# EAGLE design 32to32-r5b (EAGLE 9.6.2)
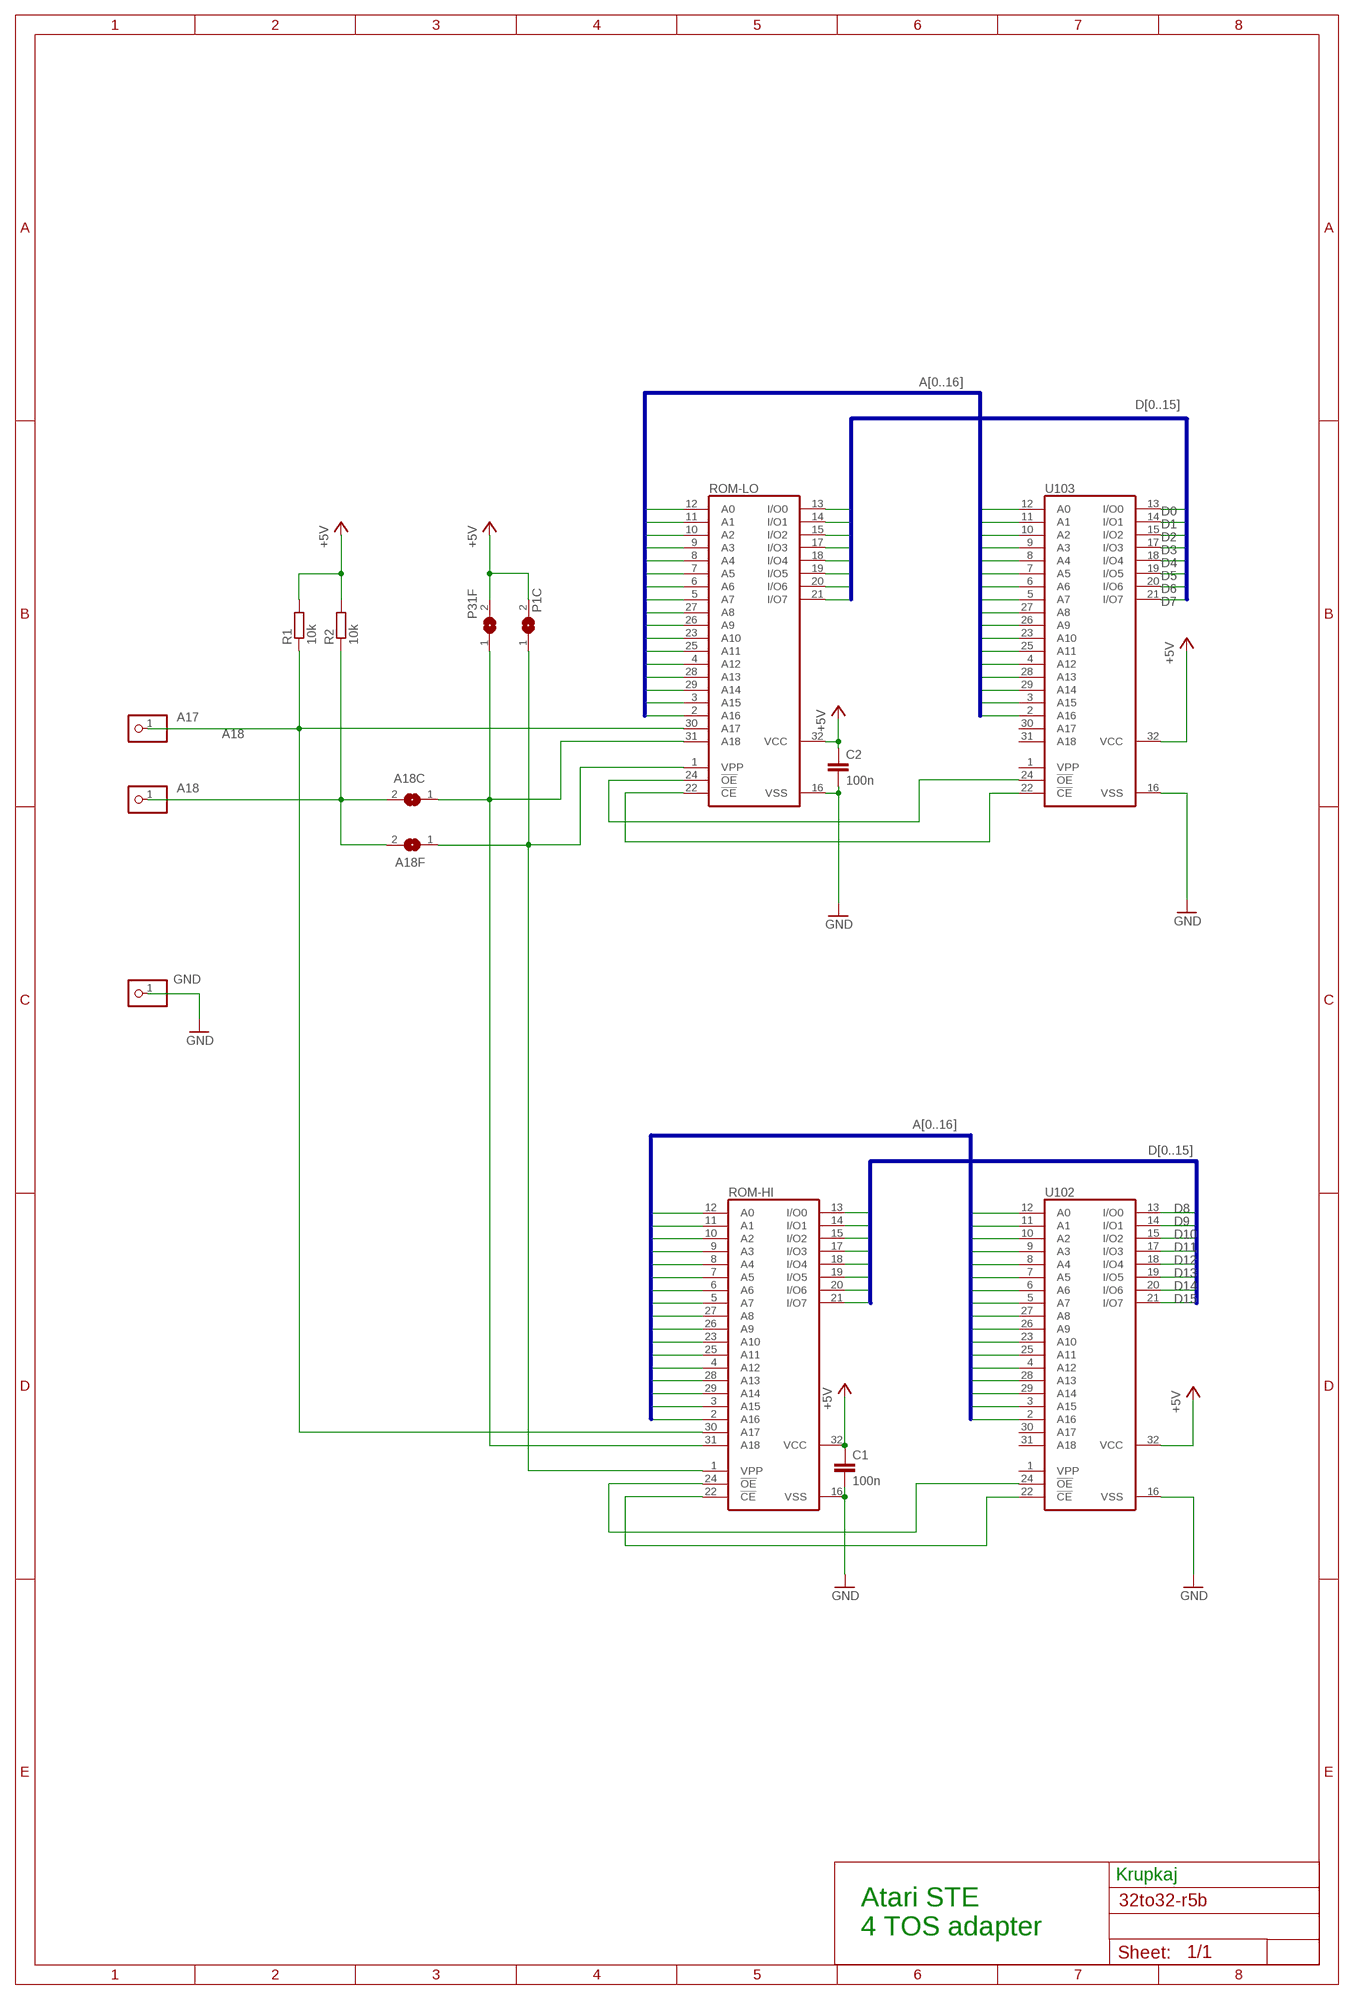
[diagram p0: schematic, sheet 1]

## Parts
A17  PINHD-1X1  [1X01]
A18  PINHD-1X1  [1X01]
A18C  SJ  [SJ]
A18F  SJ  [SJ]
C1  100n  C-EUC0805K  [C0805K]
C2  100n  C-EUC0805K  [C0805K]
GND  PINHD-1X1  [1X01]
P1C  SJ  [SJ]
P31F  SJ  [SJ]
R1  10k  R-EU_R0805  [R0805]
R2  10k  R-EU_R0805  [R0805]
ROM-HI  27C4001G  [DIL32]
ROM-LO  27C4001G  [DIL32]
U102  27C4001G  [DIL32]
U103  27C4001G  [DIL32]

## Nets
+5V: C1.1 C2.1 P1C.2 P31F.2 R1.2 R2.2 ROM-HI.32(VCC) ROM-LO.32(VCC) U102.32(VCC) U103.32(VCC)
/CE: ROM-HI.22(!CE) U102.22(!CE)
/OE: ROM-HI.24(!OE) U102.24(!OE)
A0: ROM-HI.12(A0) ROM-LO.12(A0) U102.12(A0) U103.12(A0)
A1: ROM-HI.11(A1) ROM-LO.11(A1) U102.11(A1) U103.11(A1)
A2: ROM-HI.10(A2) ROM-LO.10(A2) U102.10(A2) U103.10(A2)
A3: ROM-HI.9(A3) ROM-LO.9(A3) U102.9(A3) U103.9(A3)
A4: ROM-HI.8(A4) ROM-LO.8(A4) U102.8(A4) U103.8(A4)
A5: ROM-HI.7(A5) ROM-LO.7(A5) U102.7(A5) U103.7(A5)
A6: ROM-HI.6(A6) ROM-LO.6(A6) U102.6(A6) U103.6(A6)
A7: ROM-HI.5(A7) ROM-LO.5(A7) U102.5(A7) U103.5(A7)
A8: ROM-HI.27(A8) ROM-LO.27(A8) U102.27(A8) U103.27(A8)
A9: ROM-HI.26(A9) ROM-LO.26(A9) U102.26(A9) U103.26(A9)
A10: ROM-HI.23(A10) ROM-LO.23(A10) U102.23(A10) U103.23(A10)
A11: ROM-HI.25(A11) ROM-LO.25(A11) U102.25(A11) U103.25(A11)
A12: ROM-HI.4(A12) ROM-LO.4(A12) U102.4(A12) U103.4(A12)
A13: ROM-HI.28(A13) ROM-LO.28(A13) U102.28(A13) U103.28(A13)
A14: ROM-HI.29(A14) ROM-LO.29(A14) U102.29(A14) U103.29(A14)
A15: ROM-HI.3(A15) ROM-LO.3(A15) U102.3(A15) U103.3(A15)
A16: ROM-HI.2(A16) ROM-LO.2(A16) U102.2(A16) U103.2(A16)
A17: A17.1 R1.1 ROM-HI.30(A17) ROM-LO.30(A17)
A18: A18.1 A18C.2 A18F.2 R2.1
D0: ROM-LO.13(I/O0) U103.13(I/O0)
D1: ROM-LO.14(I/O1) U103.14(I/O1)
D2: ROM-LO.15(I/O2) U103.15(I/O2)
D3: ROM-LO.17(I/O3) U103.17(I/O3)
D4: ROM-LO.18(I/O4) U103.18(I/O4)
D5: ROM-LO.19(I/O5) U103.19(I/O5)
D6: ROM-LO.20(I/O6) U103.20(I/O6)
D7: ROM-LO.21(I/O7) U103.21(I/O7)
D8: ROM-HI.13(I/O0) U102.13(I/O0)
D9: ROM-HI.14(I/O1) U102.14(I/O1)
D10: ROM-HI.15(I/O2) U102.15(I/O2)
D11: ROM-HI.17(I/O3) U102.17(I/O3)
D12: ROM-HI.18(I/O4) U102.18(I/O4)
D13: ROM-HI.19(I/O5) U102.19(I/O5)
D14: ROM-HI.20(I/O6) U102.20(I/O6)
D15: ROM-HI.21(I/O7) U102.21(I/O7)
GND: C1.2 C2.2 GND.1 ROM-HI.16(VSS) ROM-LO.16(VSS) U102.16(VSS) U103.16(VSS)
N$1: A18C.1 P31F.1 ROM-HI.31(A18) ROM-LO.31(A18)
N$2: ROM-LO.22(!CE) U103.22(!CE)
N$3: ROM-LO.24(!OE) U103.24(!OE)
VPP: A18F.1 P1C.1 ROM-HI.1(VPP) ROM-LO.1(VPP)
Unconnected: U102.1(VPP) U102.30(A17) U102.31(A18) U103.1(VPP) U103.30(A17) U103.31(A18)

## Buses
D[0..15]
A[0..16]

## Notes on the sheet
- Krupkaj
- Atari STE
  4 TOS adapter

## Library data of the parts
A17 A18 GND = pinhead:PINHD-1X1: PIN HEADER
A18C A18F P1C P31F = jumper:SJ: SMD solder JUMPER
C1 C2 = rcl:C-EU: CAPACITOR, European symbol
R1 R2 = rcl:R-EU_: RESISTOR, European symbol
ROM-HI ROM-LO U102 U103 = memory-hitachi:27C4001G: MEMORY; OC_FARNELL: unknown; OC_NEWARK: unknown

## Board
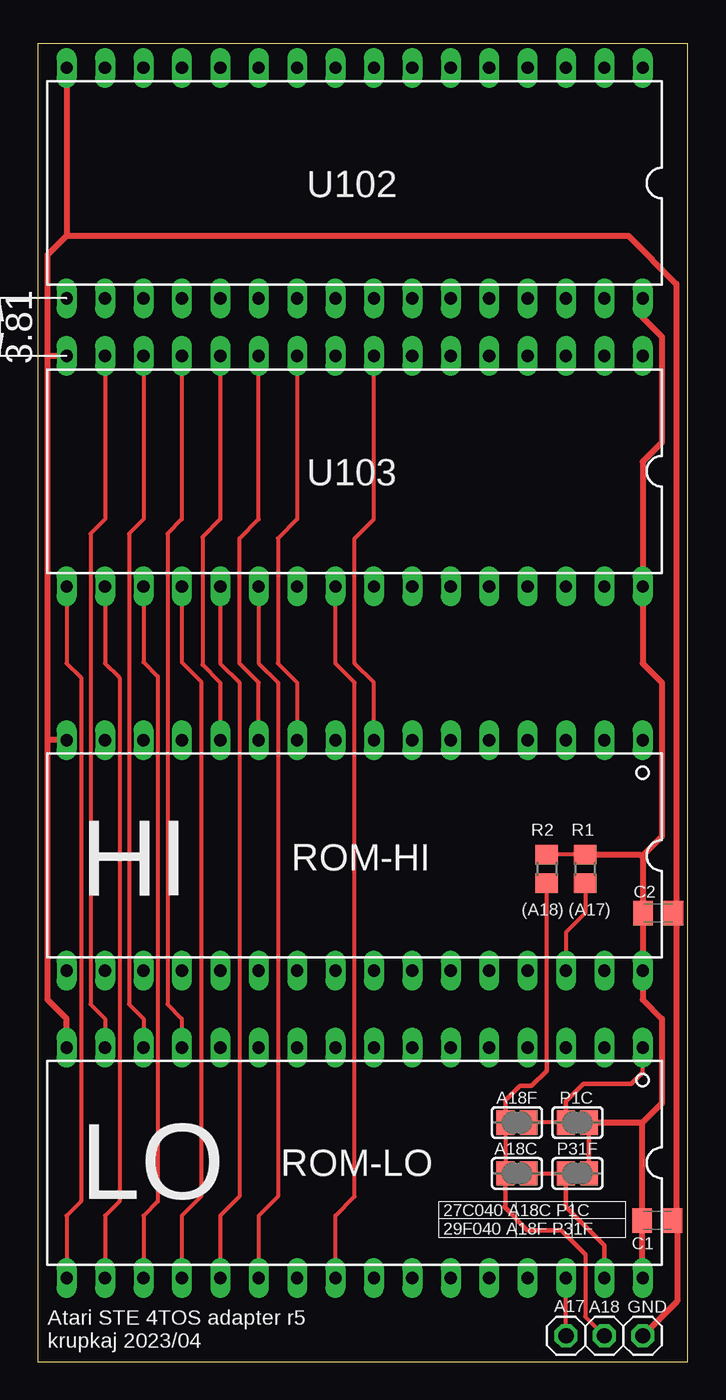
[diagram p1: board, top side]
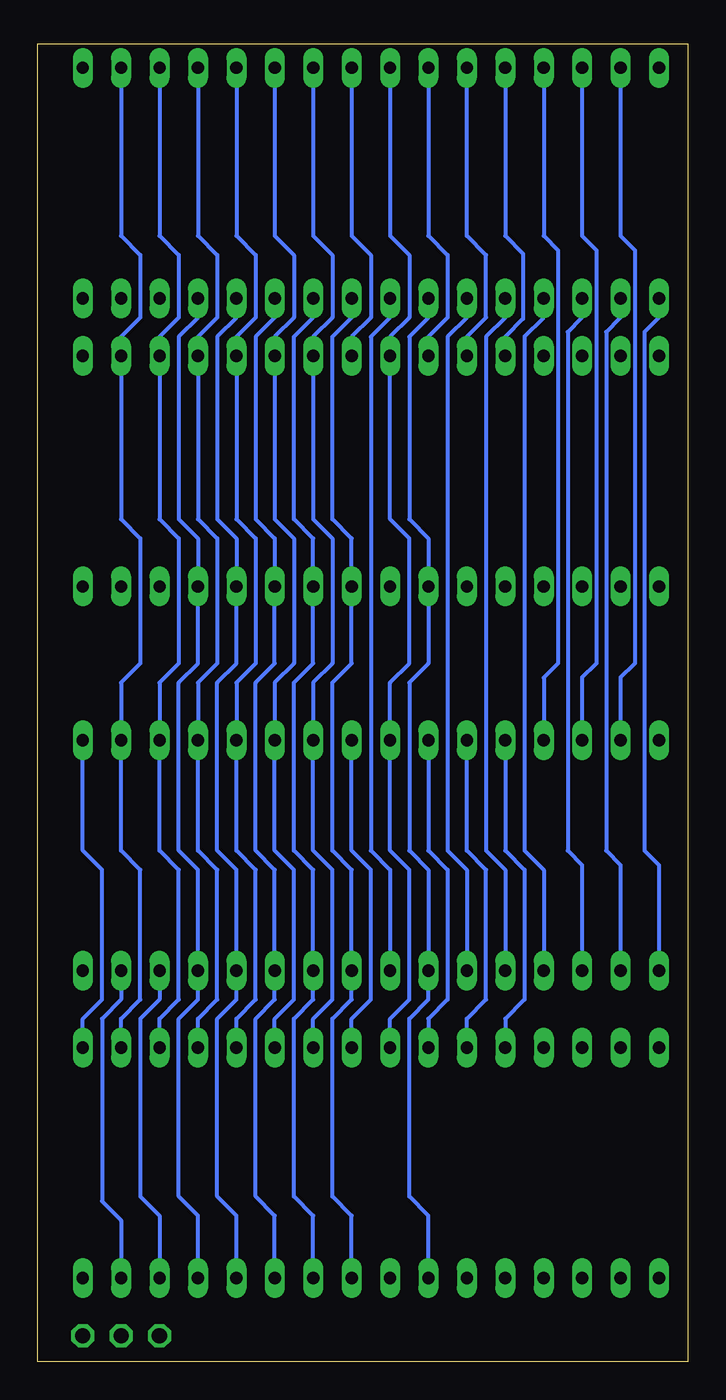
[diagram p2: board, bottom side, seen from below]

Size 42.98 x 87.11 mm. Coordinates in mm from the lower left corner, seen from the top.
Outline: 0,0 42.98,0 42.98,87.11 0,87.11 0,0
Copper layers (1*16): Top 0.035mm / dielectric 1.5mm / Bottom 0.035mm
Design rules "SeeedStudio_2layer_DRU_no_angle_20140221": minimum track width 6mil, minimum drill 12mil, track to track 6mil, track to pad 6mil, pad to pad 6mil, via to via 6mil, smd to smd 0mil, copper to edge 10mil, drill to drill 10mil, minimum pad ring 10mil, minimum via ring 6mil, stop-mask expansion 2mil, vias tented up to drill 100mil, thermal gap 10mil

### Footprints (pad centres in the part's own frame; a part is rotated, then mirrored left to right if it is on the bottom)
1X01 = drill 1.016 octagon: 1 0,0
SJ = smd 1.168 x 1.6: 1 -0.762,0; 2 0.762,0
C0805K = smd 1.3 x 1.6: 1 -1,0; 2 1,0
R0805 = smd 1.3 x 1.5: 1 -0.95,0; 2 0.95,0
DIL32 = drill 0.813 long: 1 -19.05,-7.62; 2 -16.51,-7.62; 3 -13.97,-7.62; 4 -11.43,-7.62; 5 -8.89,-7.62; 6 -6.35,-7.62; 7 -3.81,-7.62; 8 -1.27,-7.62; 9 1.27,-7.62; 10 3.81,-7.62; 11 6.35,-7.62; 12 8.89,-7.62; 13 11.43,-7.62; 14 13.97,-7.62; 15 16.51,-7.62; 16 19.05,-7.62; 17 19.05,7.62; 18 16.51,7.62; 19 13.97,7.62; 20 11.43,7.62; 21 8.89,7.62; 22 6.35,7.62; 23 3.81,7.62; 24 1.27,7.62; 25 -1.27,7.62; 26 -3.81,7.62; 27 -6.35,7.62; 28 -8.89,7.62; 29 -11.43,7.62; 30 -13.97,7.62; 31 -16.51,7.62; 32 -19.05,7.62

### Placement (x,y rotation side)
A17  34.92,1.71 0 top
A18  37.47,1.71 0 top
A18C  31.69,12.45 180 top
A18F  31.69,15.81 180 top
C1  40.96,9.33 0 top
C2  41.02,29.65 0 top
GND  40.01,1.71 0 top
P1C  35.69,15.81 0 top
P31F  35.69,12.45 0 top
R1  36.2,32.58 90 top
R2  33.66,32.58 90 top
ROM-HI  20.96,33.46 180 top
ROM-LO  20.96,13.14 180 top
U102  20.96,77.91 180 top
U103  20.96,58.86 180 top

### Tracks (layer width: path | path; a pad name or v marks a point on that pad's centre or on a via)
+5V
  Top 0.254: R2.2 R1.2 36.2,33.48
  Top 0.305: P1C.2 P31F.2
  Top 0.406: U102.32 40.01,69.02 41.28,67.75 41.28,60.77 40.01,59.5 U103.32 40.01,46.16 41.28,44.89 41.28,34.73 40.02,33.48 40.02,33.34 | 40.02,33.34 C2.1 40.02,25.86 ROM-HI.32 40.01,23.94 41.28,22.67 41.28,17.08 39.96,15.76 | 36.32,12.57 P31F.2 36.85,12.45 | ROM-LO.32 39.96,5.57 C1.1 39.96,15.76 | R1.2 39.83,33.53 40.02,33.34 | P1C.2 39.91,15.81 39.96,15.76
/CE
  Bottom 0.254: ROM-HI.22 14.61,32.51 15.88,33.78 15.88,67.75 14.61,69.02 U102.22
/OE
  Bottom 0.254: U102.24 19.68,69.02 20.96,67.75 20.96,33.78 19.68,32.51 ROM-HI.24
A0
  Top 0.254: U103.12 12.07,55.69 10.88,54.51 10.88,46.08 12.07,44.89 ROM-HI.12
  Bottom 0.254: U102.12 12.07,74.42 10.88,73.24 10.88,68.94 12.07,67.75 U103.12 | ROM-HI.12 12.07,33.78 10.79,32.51 10.79,23.94 12.07,22.67 ROM-LO.12
A1
  Top 0.254: ROM-HI.11 14.61,44.89 13.34,46.16 13.34,54.42 14.61,55.69 U103.11
  Bottom 0.254: ROM-LO.11 14.61,22.67 13.34,23.94 13.34,32.51 14.61,33.78 ROM-HI.11 | U103.11 14.61,67.75 13.34,69.02 13.34,73.15 14.61,74.42 U102.11
A2
  Top 0.254: U103.10 17.14,55.69 15.88,54.42 15.88,46.16 17.14,44.89 ROM-HI.10
  Bottom 0.254: U102.10 17.14,74.42 15.88,73.15 15.88,69.02 17.14,67.75 U103.10 | ROM-HI.10 17.14,33.78 15.88,32.51 15.88,23.94 17.14,22.67 ROM-LO.10
A3
  Bottom 0.254: U102.9 19.68,74.42 18.42,73.15 18.42,69.02 19.68,67.75 U103.9 19.68,55.69 18.42,54.42 18.42,46.16 19.68,44.89 ROM-HI.9 19.68,33.78 18.42,32.51 18.42,23.94 19.68,22.67 ROM-LO.9
A4
  Top 0.254: ROM-HI.8 22.22,44.89 20.96,46.16 20.96,54.42 22.22,55.69 U103.8
  Bottom 0.254: U102.8 22.22,74.42 20.96,73.15 20.96,69.02 22.22,67.75 U103.8 | ROM-LO.8 22.22,22.67 20.96,23.94 20.96,32.51 22.22,33.78 ROM-HI.8
A5
  Bottom 0.254: U102.7 24.77,74.42 23.5,73.15 23.5,69.02 24.77,67.75 U103.7 24.77,55.69 23.5,54.42 23.5,46.16 24.77,44.89 ROM-HI.7 24.77,33.78 23.5,32.51 23.5,23.94 24.77,22.67 ROM-LO.7
A6
  Bottom 0.254: U102.6 27.31,74.42 26.04,73.15 26.04,69.02 27.31,67.75 U103.6 27.31,55.69 26.04,54.42 26.04,46.16 27.31,44.89 ROM-HI.6 27.31,33.78 26.04,32.51 26.04,23.94 27.31,22.67 ROM-LO.6
A7
  Bottom 0.254: U102.5 29.85,74.42 28.57,73.15 28.57,69.02 29.85,67.75 U103.5 29.85,55.69 28.57,54.42 28.57,46.16 29.85,44.89 ROM-HI.5 29.85,33.78 28.57,32.51 28.57,23.94 29.85,22.67 ROM-LO.5
A8
  Bottom 0.254: ROM-LO.27 27.31,9.65 28.57,10.92 28.57,22.67 27.31,23.94 ROM-HI.27 27.31,32.51 28.57,33.78 28.57,44.89 27.31,46.16 U103.27 27.31,54.42 28.57,55.69 28.57,67.75 27.31,69.02 U102.27
A9
  Bottom 0.254: ROM-LO.26 24.77,9.65 26.04,10.92 26.04,22.67 24.77,23.94 ROM-HI.26 24.77,32.51 26.04,33.78 26.04,44.89 24.77,46.16 U103.26 24.77,54.42 26.04,55.69 26.04,67.75 24.77,69.02 U102.26
A10
  Bottom 0.254: ROM-LO.23 17.14,9.65 18.42,10.92 18.42,22.67 17.14,23.94 ROM-HI.23 17.14,32.51 18.42,33.78 18.42,44.89 17.14,46.16 U103.23 17.14,54.42 18.42,55.69 18.42,67.75 17.14,69.02 U102.23
A11
  Bottom 0.254: ROM-LO.25 22.22,9.65 23.5,10.92 23.5,22.67 22.22,23.94 ROM-HI.25 22.22,32.51 23.5,33.78 23.5,44.89 22.22,46.16 U103.25 22.22,54.42 23.5,55.69 23.5,67.75 22.22,69.02 U102.25
A12
  Bottom 0.254: U102.4 32.39,74.42 31.11,73.15 31.11,69.02 32.39,67.75 U103.4 32.39,55.69 31.11,54.42 31.11,46.16 32.39,44.89 ROM-HI.4 32.39,33.78 31.11,32.51 31.11,23.94 32.39,22.67 ROM-LO.4
A13
  Bottom 0.254: ROM-LO.28 29.85,9.65 31.11,10.92 31.11,22.67 29.85,23.94 ROM-HI.28 29.85,32.51 31.11,33.78 31.11,44.89 29.85,46.16 U103.28 29.85,54.42 31.11,55.69 31.11,67.75 29.85,69.02 U102.28
A14
  Bottom 0.254: ROM-LO.29 32.39,9.65 33.66,10.92 33.66,22.67 32.39,23.94 ROM-HI.29 32.39,32.51 33.66,33.78 33.66,44.89 32.39,46.16 U103.29 32.39,54.42 33.66,55.69 33.66,67.75 32.39,69.02 U102.29
A15
  Bottom 0.254: U102.3 34.92,74.42 33.66,73.15 33.66,69.02 34.92,67.75 U103.3 34.92,55.69 33.66,54.42 33.66,46.16 34.92,44.89 ROM-HI.3 34.92,33.78 33.66,32.51 33.66,23.94 34.92,22.67 ROM-LO.3
A16
  Bottom 0.254: U102.2 37.47,74.42 36.2,73.15 36.2,69.02 37.47,67.75 U103.2 37.47,55.69 36.2,54.42 36.2,46.16 37.47,44.89 ROM-HI.2 37.47,33.78 36.2,32.51 36.2,23.94 37.47,22.67 ROM-LO.2
A17
  Top 0.254: A17.1 ROM-LO.30 | R1.1 36.2,29.65 34.92,28.38 ROM-HI.30
  Bottom 0.254: ROM-HI.30 34.92,23.94 36.2,22.67 36.2,10.92 34.92,9.65 ROM-LO.30
A18
  Top 0.254: A18F.2 A18C.2 | 36.2,7.11 36.2,2.98 A18.1 | 33.66,19.81 R2.1
  Top 0.305: A18F.2 30.92,17.27 31.88,18.22 32.64,18.22 33.66,19.24 33.66,19.81 | A18C.2 30.92,10.29 30.86,10.22 32.39,8.7 34.61,8.7 36.2,7.11
D0
  Top 0.254: U103.13 9.53,55.69 8.57,54.74 8.57,23.62 9.53,22.67 ROM-LO.13
D1
  Top 0.254: U103.14 6.98,55.69 6.03,54.74 6.03,23.62 6.98,22.67 ROM-LO.14
D2
  Top 0.254: U103.15 4.45,55.69 3.49,54.74 3.49,23.62 4.45,22.67 ROM-LO.15
D3
  Top 0.254: U103.17 1.91,46.16 2.86,45.21 2.86,10.6 1.91,9.65 ROM-LO.17
D4
  Top 0.254: U103.18 4.45,46.16 5.4,45.21 5.4,10.6 4.45,9.65 ROM-LO.18
D5
  Top 0.254: U103.19 6.98,46.25 7.93,45.31 7.93,10.59 6.98,9.65 ROM-LO.19
D6
  Top 0.254: U103.20 9.53,46.25 10.79,44.98 10.79,10.92 9.53,9.65 ROM-LO.20
D7
  Top 0.254: U103.21 12.07,46.16 13.34,44.89 13.34,10.92 12.07,9.65 ROM-LO.21
D8
  Bottom 0.254: U102.13 9.53,74.42 8.57,73.47 8.57,46.16 9.53,45.21 ROM-HI.13
D9
  Bottom 0.254: U102.14 6.98,74.42 6.03,73.47 6.03,46.16 6.98,45.21 ROM-HI.14
D10
  Bottom 0.254: U102.15 4.45,74.42 3.49,73.47 3.49,46.16 4.45,45.21 ROM-HI.15
D11
  Bottom 0.254: U102.17 1.91,69.02 2.86,68.07 2.86,33.78 1.91,32.83 ROM-HI.17
D12
  Bottom 0.254: U102.18 4.45,69.02 5.4,68.07 5.4,33.78 4.45,32.83 ROM-HI.18
D13
  Bottom 0.254: U102.19 6.98,69.02 7.94,68.07 7.94,33.78 6.98,32.83 ROM-HI.19
D14
  Bottom 0.254: U102.20 9.53,69.02 10.79,67.75 10.79,33.78 9.53,32.51 ROM-HI.20
D15
  Bottom 0.254: U102.21 12.07,69.02 13.34,67.75 13.34,33.78 12.07,32.51 ROM-HI.21
GND
  Top 0.406: U102.16 1.91,74.42 | 1.91,74.42 0.64,73.15 0.64,66.48 | U103.16 0.64,66.48 | 0.64,66.48 0.64,41.08 | ROM-HI.16 0.64,41.08 | ROM-LO.16 1.91,22.67 0.64,23.94 0.64,41.08 | 1.91,74.42 39.05,74.42 42.23,71.25 42.23,29.86 C2.2 42.21,29.46 42.21,9.59 C1.2 42.28,9.02 42.28,3.98 GND.1
N$1
  Top 0.254: A18C.1 P31F.1
  Top 0.305: P31F.1 34.92,10.22 37.47,7.68 ROM-LO.31
  Bottom 0.254: ROM-HI.31 37.47,23.94 38.73,22.67 38.73,10.6 37.47,9.33 ROM-LO.31
N$2
  Top 0.254: U103.22 14.61,46.16 15.88,44.89 15.88,10.92 14.61,9.65 ROM-LO.22
N$3
  Top 0.254: ROM-LO.24 19.68,9.65 20.96,10.92 20.96,44.89 19.68,46.16 U103.24
VPP
  Top 0.254: P1C.1 A18F.1 | 40.01,19.11 ROM-LO.1
  Top 0.305: P1C.1 34.92,17.21 36.07,18.35 39.24,18.35 40.01,19.11
  Bottom 0.254: ROM-HI.1 40.01,33.78 38.73,32.51 38.73,23.94 40.01,22.67 ROM-LO.1

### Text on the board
tPlace: Atari STE 4TOS adapter r5 / krupkaj 2023/04
tNames: HI | (A18) (A17) | LO | 27C040 A18C P1C / 29F040 A18F P31F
